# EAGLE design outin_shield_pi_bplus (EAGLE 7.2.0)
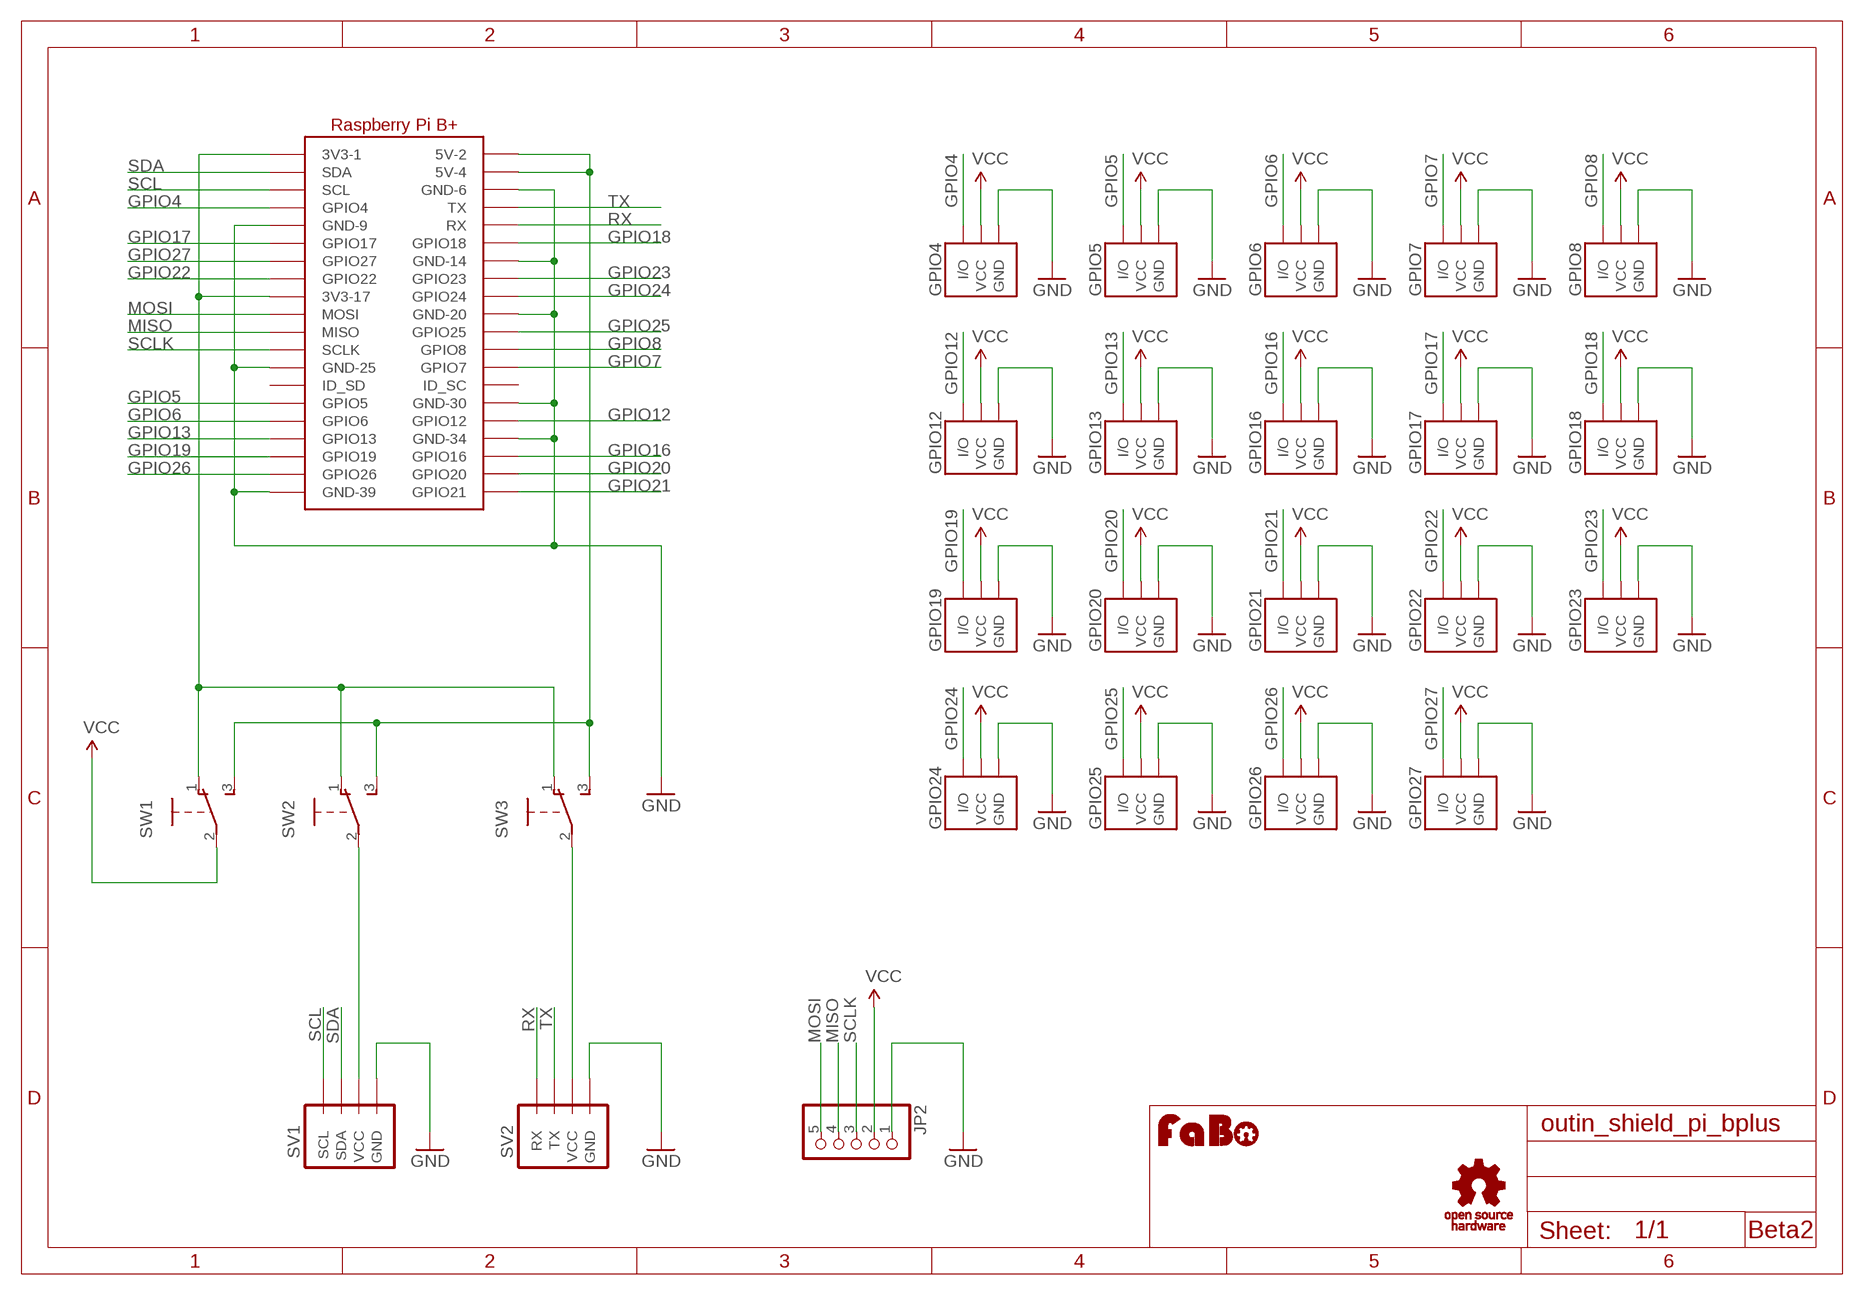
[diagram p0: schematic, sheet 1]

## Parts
GPIO4  IO_PIN-3PIN  [1X3-SNEAKY]
GPIO5  IO_PIN-3PIN  [1X3-SNEAKY]
GPIO6  IO_PIN-3PIN  [1X3-SNEAKY]
GPIO7  IO_PIN-3PIN  [1X3-SNEAKY]
GPIO8  IO_PIN-3PIN  [1X3-SNEAKY]
GPIO12  IO_PIN-3PIN  [1X3-SNEAKY]
GPIO13  IO_PIN-3PIN  [1X3-SNEAKY]
GPIO16  IO_PIN-3PIN  [1X3-SNEAKY]
GPIO17  IO_PIN-3PIN  [1X3-SNEAKY]
GPIO18  IO_PIN-3PIN  [1X3-SNEAKY]
GPIO19  IO_PIN-3PIN  [1X3-SNEAKY]
GPIO20  IO_PIN-3PIN  [1X3-SNEAKY]
GPIO21  IO_PIN-3PIN  [1X3-SNEAKY]
GPIO22  IO_PIN-3PIN  [1X3-SNEAKY]
GPIO23  IO_PIN-3PIN  [1X3-SNEAKY]
GPIO24  IO_PIN-3PIN  [1X3-SNEAKY]
GPIO25  IO_PIN-3PIN  [1X3-SNEAKY]
GPIO26  IO_PIN-3PIN  [1X3-SNEAKY]
GPIO27  IO_PIN-3PIN  [1X3-SNEAKY]
JP2  PINHD-1X5  [1X05]
SV1  BRICK_I2C_CONNECTOR  [BRICK_I2C_CONNECTOR]
SV2  BRICK_SERIAL_CONNECTOR  [BRICK_SERIAL_CONNECTOR]
SW1  SWITCH-SLIDE-EG1218  [EG1218]
SW2  SWITCH-SLIDE-EG1218  [EG1218]
SW3  SWITCH-SLIDE-EG1218  [EG1218]
U1  RASPBERRY_PI_B+  [RASPBERRY_PI_B+]
U$14  LOGO_FABO-M  [LOGO_FABO_M]
U$15  LOGO_OSHW_T-M  [LOGO_OSHW_T_M]

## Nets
3V3: SW1.1 SW2.1 SW3.1 U1.1(3V3-1) U1.17(3V3-17)
5V: SW1.3 SW2.3 SW3.3 U1.2(5V-2) U1.4(5V-4)
GND: GPIO4.1(GND) GPIO5.1(GND) GPIO6.1(GND) GPIO7.1(GND) GPIO8.1(GND) GPIO12.1(GND) GPIO13.1(GND) GPIO16.1(GND) GPIO17.1(GND) GPIO18.1(GND) GPIO19.1(GND) GPIO20.1(GND) GPIO21.1(GND) GPIO22.1(GND) GPIO23.1(GND) GPIO24.1(GND) GPIO25.1(GND) GPIO26.1(GND) GPIO27.1(GND) JP2.1 SV1.GND SV2.GND U1.6(GND-6) U1.9(GND-9) U1.14(GND-14) U1.20(GND-20) U1.25(GND-25) U1.30(GND-30) U1.34(GND-34) U1.39(GND-39)
GPIO4: GPIO4.3(I/O) U1.7(GPIO4)
GPIO5: GPIO5.3(I/O) U1.29(GPIO5)
GPIO6: GPIO6.3(I/O) U1.31(GPIO6)
GPIO7: GPIO7.3(I/O) U1.26(GPIO7)
GPIO8: GPIO8.3(I/O) U1.24(GPIO8)
GPIO12: GPIO12.3(I/O) U1.32(GPIO12)
GPIO13: GPIO13.3(I/O) U1.33(GPIO13)
GPIO16: GPIO16.3(I/O) U1.36(GPIO16)
GPIO17: GPIO17.3(I/O) U1.11(GPIO17)
GPIO18: GPIO18.3(I/O) U1.12(GPIO18)
GPIO19: GPIO19.3(I/O) U1.35(GPIO19)
GPIO20: GPIO20.3(I/O) U1.38(GPIO20)
GPIO21: GPIO21.3(I/O) U1.40(GPIO21)
GPIO22: GPIO22.3(I/O) U1.15(GPIO22)
GPIO23: GPIO23.3(I/O) U1.16(GPIO23)
GPIO24: GPIO24.3(I/O) U1.18(GPIO24)
GPIO25: GPIO25.3(I/O) U1.22(GPIO25)
GPIO26: GPIO26.3(I/O) U1.37(GPIO26)
GPIO27: GPIO27.3(I/O) U1.13(GPIO27)
I2C_PWR: SV1.VCC SW2.2
MISO: JP2.4 U1.21(MISO)
MOSI: JP2.5 U1.19(MOSI)
RX: SV2.RX U1.10(RX)
SCL: SV1.SCL U1.5(SCL)
SCLK: JP2.3 U1.23(SCLK)
SDA: SV1.SDA U1.3(SDA)
SERIAL_PWR: SV2.VCC SW3.2
TX: SV2.TX U1.8(TX)
VCC: GPIO4.2(VCC) GPIO5.2(VCC) GPIO6.2(VCC) GPIO7.2(VCC) GPIO8.2(VCC) GPIO12.2(VCC) GPIO13.2(VCC) GPIO16.2(VCC) GPIO17.2(VCC) GPIO18.2(VCC) GPIO19.2(VCC) GPIO20.2(VCC) GPIO21.2(VCC) GPIO22.2(VCC) GPIO23.2(VCC) GPIO24.2(VCC) GPIO25.2(VCC) GPIO26.2(VCC) GPIO27.2(VCC) JP2.2 SW1.2
Unconnected: U1.27(ID_SD) U1.28(ID_SC)

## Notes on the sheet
- Beta2

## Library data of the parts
GPIO4-GPIO8 GPIO12 GPIO13 GPIO16-GPIO27 = Gclue:IO_PIN
JP2 = pinhead:PINHD-1X5: PIN HEADER
SV1 = Gclue:BRICK_I2C_CONNECTOR: Brick Connector female for OUT/IN Shield
SV2 = Gclue:BRICK_SERIAL_CONNECTOR
SW1-SW3 = Gclue:SWITCH-SLIDE
U1 = Gclue:RASPBERRY_PI_B+
U$14 = FaBo:LOGO_FABO
U$15 = Gclue:LOGO_OSHW_T

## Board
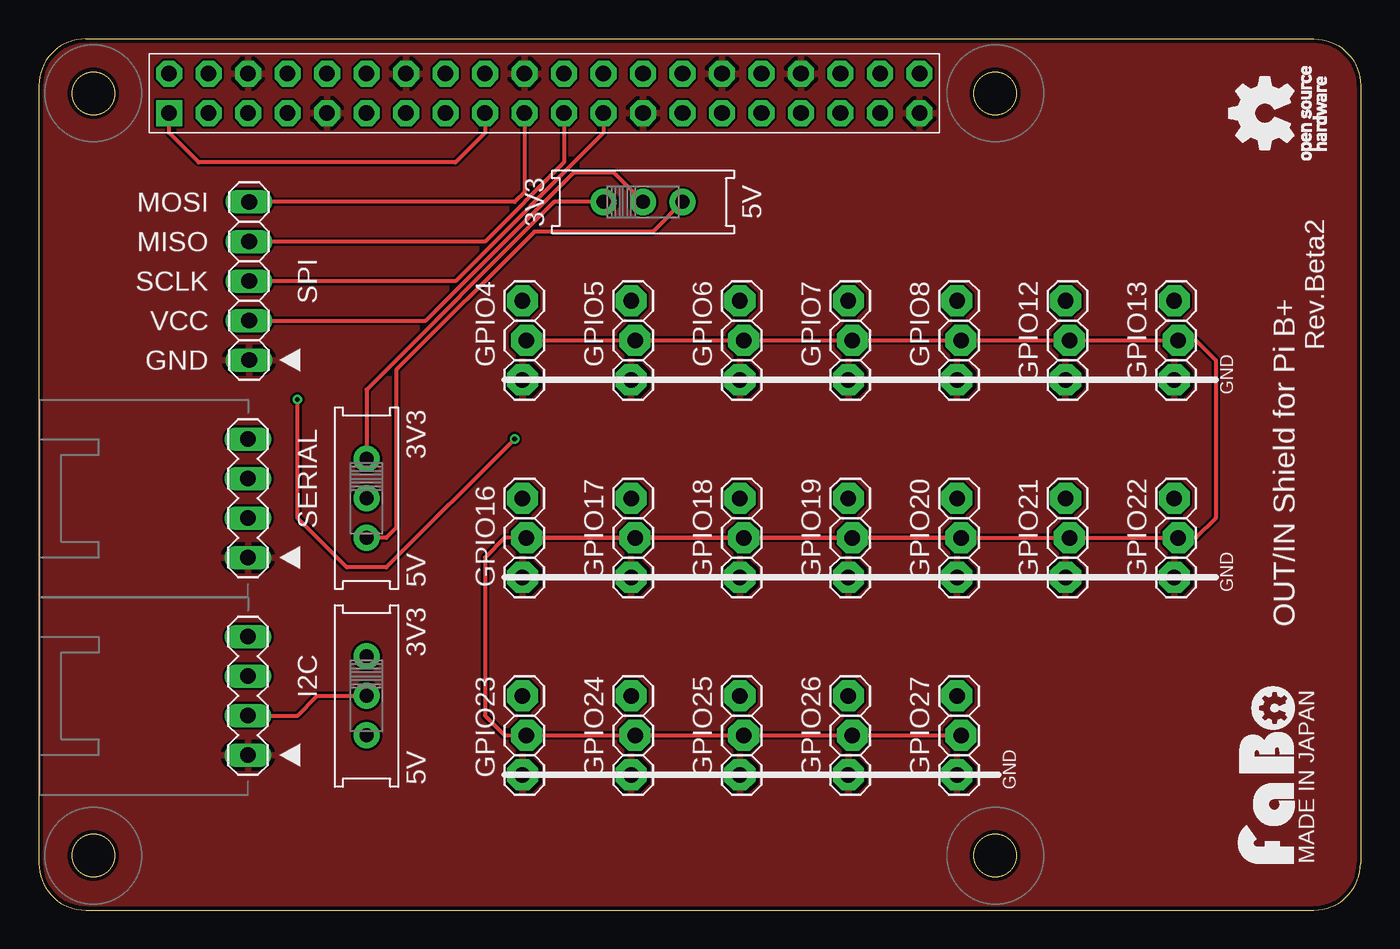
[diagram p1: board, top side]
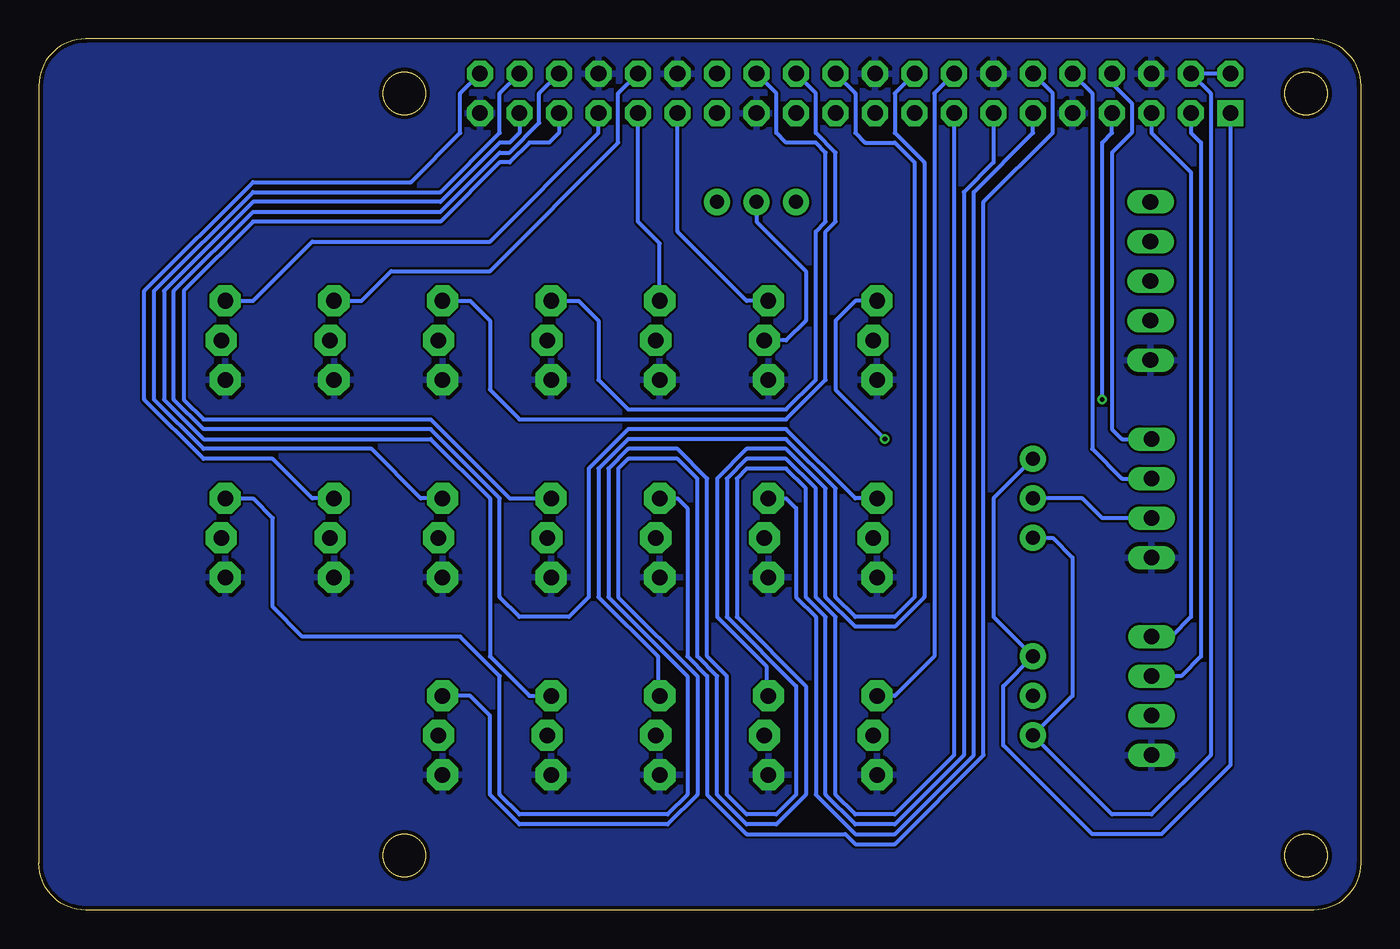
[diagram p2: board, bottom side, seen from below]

Size 85 x 56 mm. Coordinates in mm from the lower left corner, seen from the top.
Copper layers (1*16): Top 0.035mm / dielectric 1.5mm / Bottom 0.035mm
Design rules "Elecrow_2-layer_eagle_rule": minimum track width 6mil, minimum drill 12mil, track to track 6mil, track to pad 6mil, pad to pad 6mil, via to via 6mil, smd to smd 0mil, copper to edge 10mil, drill to drill 10mil, minimum pad ring 10mil, minimum via ring 6mil, stop-mask expansion 2mil, vias tented up to drill 100mil, thermal gap 10mil

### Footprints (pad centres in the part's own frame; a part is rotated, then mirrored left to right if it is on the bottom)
1X3-SNEAKY = drill 1 pad 2 octagon: 1 -2.54,0.127; 2 0,-0.127; 3 2.54,0.127
1X05 = drill 1.016 long: 1 -5.08,0; 2 -2.54,0; 3 0,0; 4 2.54,0; 5 5.08,0
BRICK_I2C_CONNECTOR = drill 1 long: GND -3.81,0; SCL 3.81,0; SDA 1.27,0; VCC -1.27,0
BRICK_SERIAL_CONNECTOR = drill 1 long: GND -3.81,0; RX 1.27,0; TX 3.81,0; VCC -1.27,0
EG1218 = drill 0.9 pad 1.676: 1 -2.54,0; 2 0,0; 3 2.54,0
RASPBERRY_PI_B+ = drill 1 pad 1.676 square: 1 8.89,52.07 | drill 1 pad 1.676 octagon: 2 8.89,54.61; 3 11.43,52.07; 4 11.43,54.61; 5 13.97,52.07; 6 13.97,54.61; 7 16.51,52.07; 8 16.51,54.61; 9 19.05,52.07; 10 19.05,54.61; 11 21.59,52.07; 12 21.59,54.61; 13 24.13,52.07; 14 24.13,54.61; 15 26.67,52.07; 16 26.67,54.61; 17 29.21,52.07; 18 29.21,54.61; 19 31.75,52.07; 20 31.75,54.61; 21 34.29,52.07; 22 34.29,54.61; 23 36.83,52.07; 24 36.83,54.61; 25 39.37,52.07; 26 39.37,54.61; 27 41.91,52.07; 28 41.91,54.61; 29 44.45,52.07; 30 44.45,54.61; 31 46.99,52.07; 32 46.99,54.61; 33 49.53,52.07; 34 49.53,54.61; 35 52.07,52.07; 36 52.07,54.61; 37 54.61,52.07; 38 54.61,54.61; 39 57.15,52.07; 40 57.15,54.61

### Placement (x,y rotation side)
GPIO4  31.23,36.62 90 top
GPIO5  38.21,36.62 90 top
GPIO6  45.2,36.62 90 top
GPIO7  52.18,36.62 90 top
GPIO8  59.17,36.62 90 top
GPIO12  66.16,36.62 90 top
GPIO13  73.14,36.62 90 top
GPIO16  31.23,23.93 90 top
GPIO17  38.21,23.93 90 top
GPIO18  45.2,23.93 90 top
GPIO19  52.18,23.93 90 top
GPIO20  59.17,23.93 90 top
GPIO21  66.16,23.93 90 top
GPIO22  73.14,23.93 90 top
GPIO23  31.23,11.22 90 top
GPIO24  38.21,11.22 90 top
GPIO25  45.2,11.22 90 top
GPIO26  52.18,11.22 90 top
GPIO27  59.17,11.22 90 top
JP2  13.52,40.43 90 top
SV1  13.45,13.77 90 top
SV2  13.45,26.46 90 top
SW1  38.85,45.51 0 top
SW2  21.07,13.77 270 top
SW3  21.07,26.46 270 top
U1  -0.52,-0.84 0 top
U$14  80.76,8.69 90 top
U$15  78.86,51.23 90 top

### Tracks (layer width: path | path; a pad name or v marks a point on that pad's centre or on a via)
3V3
  Top 0.254: SW1.1 33.13,45.51 21.07,33.45 SW3.1 | U1.17 28.69,49.96 26.79,48.05 10.28,48.05 8.37,49.96 U1.1
  Bottom 0.254: SW3.1 23.61,26.46 23.61,18.84 SW2.1 22.98,14.4 22.98,10.59 17.26,4.88 12.82,4.88 8.37,9.32 U1.1
5V
  Top 0.254: SW1.3 39.48,43.61 31.86,43.61 22.98,34.72 22.98,24.56 22.34,23.93 SW3.3
  Bottom 0.254: SW3.3 19.8,23.93 18.53,22.66 18.53,13.77 SW2.3 15.99,6.15 13.45,6.15 9.64,9.96 9.64,52.5 U1.4 U1.2
GND
  pour Bottom: -1.79,-2.11 87.11,-2.11 87.11,57.58 -1.79,57.58
  pour Top: -1.79,-2.11 87.11,-2.11 87.11,57.58 -1.79,57.58
GPIO4  (via drill 0.3)
  Top 0.254: v30.59,30.27 22.34,22.02 19.8,22.02 16.62,25.2 v16.62,32.81
  Bottom 0.254: GPIO4.3 32.5,39.16 33.77,37.89 33.77,33.45 v30.59,30.27 | v16.62,32.81 16.62,49.32 15.99,49.96 U1.7
GPIO5
  Bottom 0.254: GPIO5.3 39.48,39.16 43.93,43.61 U1.29
GPIO6
  Bottom 0.254: GPIO6.3 45.07,42.85 46.47,44.24 U1.31
GPIO7
  Bottom 0.254: GPIO7.3 50.28,39.16 49.01,37.89 49.01,34.08 47.1,32.18 36.95,32.18 35.04,34.08 35.04,43.61 34.4,44.24 34.4,48.69 35.04,49.32 36.95,49.32 37.58,49.96 37.58,52.5 U1.26
GPIO8
  Bottom 0.254: GPIO8.3 57.26,39.16 55.99,37.89 55.99,33.45 54.09,31.54 36.95,31.54 34.4,34.08 34.4,43.61 33.77,44.24 33.77,48.69 35.04,49.96 35.04,52.5 U1.24
GPIO12
  Bottom 0.254: GPIO12.3 64.25,39.16 62.34,41.07 55.99,41.07 47.74,49.32 47.74,52.5 U1.32
GPIO13
  Bottom 0.254: GPIO13.3 71.23,39.16 67.42,42.97 55.99,42.97 49.01,49.96 U1.33
GPIO16
  Bottom 0.254: GPIO16.3 32.5,26.46 36.95,30.91 47.1,30.91 49.64,28.37 49.64,20.11 50.91,18.84 54.09,18.84 55.36,20.11 55.36,26.46 59.8,30.91 74.41,30.91 76.31,32.81 76.31,39.8 71.23,44.88 59.17,44.88 55.36,48.69 54.72,48.69 52.82,50.59 52.82,52.5 U1.36
GPIO17
  Bottom 0.254: GPIO17.3 36.95,26.46 36.31,25.83 36.31,20.11 35.04,18.84 35.04,7.42 32.5,4.88 29.96,4.88 24.88,9.96 24.88,46.15 21.07,49.96 U1.11
GPIO18
  Bottom 0.254: GPIO18.3 43.93,26.46 43.29,25.83 43.29,16.3 42.02,15.04 42.02,7.42 39.48,4.88 33.13,4.88 32.5,4.24 29.96,4.24 24.25,9.96 24.25,45.51 19.8,49.96 19.8,52.5 U1.12
GPIO19
  Bottom 0.254: U1.35 51.55,49.96 52.18,49.32 53.45,49.32 54.72,48.05 55.36,48.05 59.17,44.24 71.23,44.24 75.68,39.8 75.68,32.81 74.41,31.54 59.8,31.54 54.72,26.46 GPIO19.3
GPIO20
  Bottom 0.254: GPIO20.3 60.44,26.46 63.62,29.64 74.41,29.64 77.59,32.81 77.59,39.8 71.23,46.15 59.17,46.15 55.36,49.96 55.36,52.5 U1.38
GPIO21
  Bottom 0.254: GPIO21.3 67.42,26.46 69.97,29 74.41,29 78.22,32.81 78.22,39.8 71.23,46.78 61.07,46.78 57.9,49.96 57.9,52.5 U1.40
GPIO22
  Bottom 0.254: U1.15 26.15,9.96 29.96,6.15 32.5,6.15 33.77,7.42 33.77,18.84 35.04,20.11 35.04,27.1 36.95,29 39.48,29 40.75,27.73 40.75,18.84 36.31,14.4 36.31,7.42 37.58,6.15 39.48,6.15 40.75,7.42 40.75,15.04 42.02,16.3 42.02,27.73 43.93,29.64 47.1,29.64 48.38,28.37 48.38,20.11 43.29,15.04 43.29,7.42 44.56,6.15 54.09,6.15 55.36,7.42 55.36,15.04 57.9,17.57 68.06,17.57 69.97,19.48 69.97,25.2 71.23,26.46 GPIO22.3
GPIO23
  Bottom 0.254: U1.16 27.42,52.5 27.42,16.3 29.96,13.77 GPIO23.3
GPIO24
  Bottom 0.254: U1.18 29.96,52.5 29.96,49.96 28.05,48.05 28.05,20.11 29.96,18.21 32.5,18.21 34.4,20.11 34.4,27.1 36.95,29.64 39.48,29.64 41.39,27.73 41.39,18.84 38.21,15.67 38.21,13.77 GPIO24.3
GPIO25
  Bottom 0.254: U1.22 32.5,52.5 32.5,49.96 31.86,49.32 29.96,49.32 28.69,48.05 28.69,20.11 29.96,18.84 32.5,18.84 33.77,20.11 33.77,27.1 36.95,30.27 47.1,30.27 49.01,28.37 49.01,20.11 45.2,16.3 45.2,13.77 GPIO25.3
GPIO26
  Bottom 0.254: U1.37 54.09,49.96 54.72,49.32 55.36,49.32 59.17,45.51 71.23,45.51 76.95,39.8 76.95,32.81 74.41,30.27 59.8,30.27 55.99,26.46 55.99,16.3 53.45,13.77 GPIO26.3
GPIO27
  Bottom 0.254: U1.13 23.61,48.05 25.52,46.15 25.52,9.96 29.96,5.51 32.5,5.51 34.4,7.42 34.4,18.84 35.67,20.11 35.67,27.1 36.95,28.37 39.48,28.37 40.12,27.73 40.12,18.84 35.67,14.4 35.67,7.42 37.58,5.51 39.48,5.51 41.39,7.42 41.39,15.04 42.66,16.3 42.66,27.73 43.93,29 47.1,29 47.74,28.37 47.74,20.11 42.66,15.04 42.66,7.42 44.56,5.51 54.09,5.51 55.99,7.42 55.99,12.5 57.26,13.77 GPIO27.3
I2C_PWR
  Top 0.254: SV1.VCC 16.62,12.5 17.89,13.77 SW2.2
MISO
  Top 0.254: U1.21 33.77,48.05 28.69,42.97 JP2.4
MOSI
  Top 0.254: U1.19 31.23,46.15 30.59,45.51 JP2.5
RX
  Bottom 0.254: U1.10 17.26,52.5 17.26,29.64 15.36,27.73 SV2.RX
SCL
  Bottom 0.254: U1.5 13.45,49.96 10.91,47.42 10.91,18.84 12.18,17.57 SV1.SCL
SCLK
  Top 0.254: U1.23 36.31,49.96 26.79,40.43 JP2.3
SDA
  Bottom 0.254: U1.3 10.91,49.96 10.28,49.32 10.28,16.3 11.54,15.04 SV1.SDA
SERIAL_PWR
  Bottom 0.254: SV2.VCC 16.62,25.2 17.89,26.46 SW3.2
TX
  Bottom 0.254: U1.8 15.99,53.13 14.72,51.86 14.72,49.96 15.99,48.69 15.99,30.91 15.36,30.27 SV2.TX
VCC
  Top 0.254: GPIO27.2 GPIO26.2 GPIO25.2 GPIO24.2 GPIO23.2 29.96,11.22 28.69,12.5 28.69,22.66 29.96,23.93 GPIO20.2 | GPIO16.2 GPIO17.2 GPIO18.2 GPIO19.2 GPIO20.2 | GPIO20.2 GPIO21.2 GPIO22.2 74.41,23.93 75.68,25.2 75.68,35.35 74.41,36.62 GPIO4.2 GPIO5.2 GPIO6.2 GPIO7.2 GPIO8.2 GPIO12.2 GPIO13.2 | JP2.2 24.88,37.89 34.4,47.42 36.95,47.42 SW1.2
  Bottom 0.254: SW1.2 38.85,44.24 35.67,41.07 35.67,37.89 36.95,36.62 GPIO5.2

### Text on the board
tPlace: MOSI | 3V3 | 5V | MISO | SCLK | SPI | VCC | Rev.Beta2 | GND | ▲ | GND | 3V3 | SERIAL | ▲ | 5V | GND | 3V3 | OUT/IN Shield for Pi B+ | I2C | ▲ | 5V | GND | MADE IN JAPAN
